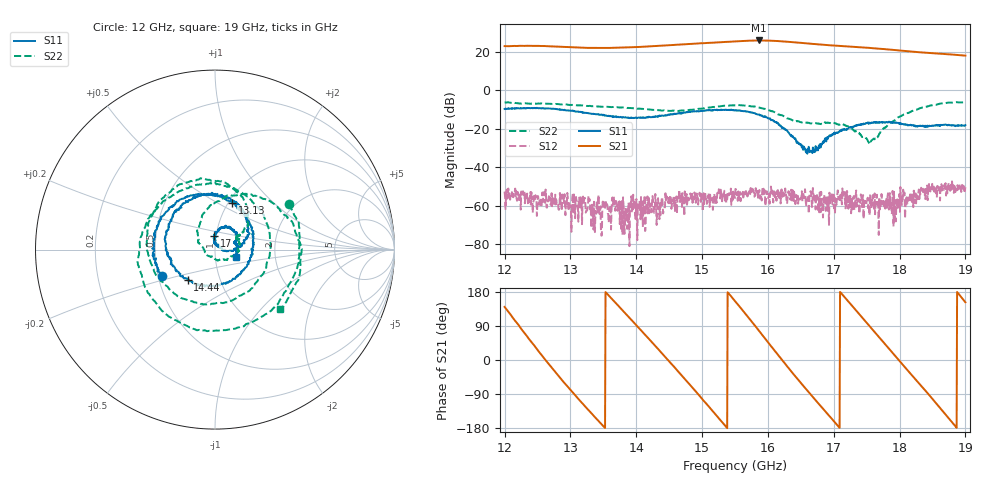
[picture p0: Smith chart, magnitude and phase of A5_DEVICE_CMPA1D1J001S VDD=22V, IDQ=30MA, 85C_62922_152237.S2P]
!Keysight Technologies,E5071C,MY46631738,B.14.03
!Date: Wed Jun 29 17:29:15 2022
!Data & Calibration Information:
!Freq	S11:SOLT2(ON)	S21:SOLT2(ON)	S12:SOLT2(ON)	S22:SOLT2(ON)
!PortZ  Port1:50+j0  Port2:50+j0
!Above PortZ is port z conversion or system Z0 setting when saving the data.
!When reading, reference impedance value at option line is always used.
# Hz S dB R 50
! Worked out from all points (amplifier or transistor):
!   1001 points, 12 GHz to 19 GHz, reference 50 ohm
!   highest |S21| = 25.9 dB at 15.86 GHz (marker M1)
!   |S21| within 3 dB of that: 14.24 GHz to 17.15 GHz (2.912 GHz wide, 18.5 % of centre)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
!   unconditionally stable (mu >= 1): start of sweep to end of sweep
!   at 13.16 GHz: K = 30.47, MAG = 23.3 dB, |S12| = -60.2 dB
!   at 15.5 GHz: K = 12.59, MAG = 26.7 dB, |S12| = -55.9 dB
!   at 19 GHz: K = 15.32, MAG = 19.3 dB, |S12| = -50.3 dB
!   S11 on the Smith chart (normalised r, x): 12 GHz: 0.53, -0.18; 13.13 GHz: 1.04, +0.59; 14.44 GHz: 0.70, -0.25; 17 GHz: 0.98, +0.15; 19 GHz: 1.26, -0.10
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1.2e10  -9.64 -153.0  23.01 140.0  -52.60 -141.3  -6.28 31.5
1.2273e10  -9.33 175.2  23.15 77.4  -54.35 172.3  -6.78 -38.1
1.2581e10  -9.29 138.0  23.06 9.2  -58.05 121.6  -6.83 -108.1
1.2875e10  -10.17 100.9  22.63 -53.9  -54.06 85.3  -7.27 -164.6
1.3127e10  -11.17 70.0  22.24 -104.1  -56.16 45.3  -7.76 158.1
1.3169e10  -11.25 65.5  22.18 -112.0  -56.38 56.0  -7.84 153.1
1.3652e10  -13.47 -1.7  22.10 157.1  -56.42 -107.1  -8.61 94.3
1.4009e10  -14.40 -58.0  22.53 90.1  -64.77 -47.8  -9.47 47.3
1.4338e10  -13.29 -111.1  23.13 27.9  -61.42 87.7  -10.29 -4.2
1.4443e10  -12.85 -131.9  23.34 7.7  -53.45 178.6  -10.45 -23.8
1.4695e10  -11.77 -168.4  23.90 -41.5  -60.54 105.6  -10.39 -75.6
1.4982e10  -10.59 151.1  24.50 -98.8  -57.95 70.3  -9.56 -136.0
1.5269e10  -10.20 115.1  24.98 -156.9  -54.34 40.9  -8.27 169.2
1.55e10  -10.38 84.5  25.45 155.4  -55.88 -26.4  -7.78 130.5
1.5864e10  -12.58 39.2  25.94 77.3  -52.43 -80.1  -8.91 75.7
1.6221e10  -19.23 -0.9  25.48 -1.5  -55.25 -156.2  -13.02 35.7
1.6669e10  -32.27 64.7  24.20 -94.9  -60.61 124.8  -17.15 29.3
1.6998e10  -22.34 94.0  23.33 -160.7  -53.07 75.9  -16.91 13.3
1.7439e10  -17.62 67.8  22.30 110.6  -55.67 25.0  -24.09 -64.2
1.7838e10  -16.20 38.2  21.23 29.9  -61.89 -93.2  -17.41 135.6
1.8398e10  -18.34 18.7  19.55 -82.0  -51.27 -48.1  -8.51 53.3
1.9e10  -18.08 -18.7  18.06 152.3  -50.31 -151.6  -6.20 -42.7
